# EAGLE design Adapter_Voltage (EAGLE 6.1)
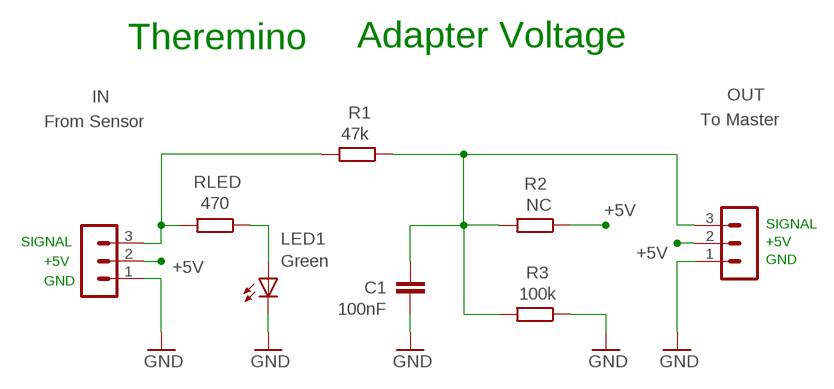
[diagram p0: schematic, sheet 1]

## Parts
C1  100nF  C-EU025-024X044  [C025-024X044]
IN  From Sensor  MA03-1N  [MA03-1]
LED1  Green  LED3MM_F  [LED3MM]
OUT  To Master  MA03-1N  [MA03-1]
R1  47k  R-EU_0204/5  [0204/5]
R2  NC  R-EU_0204/5  [0204/5]
R3  100k  R-EU_0204/5  [0204/5]
RLED  470  R-EU_0204/5  [0204/5]

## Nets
+5V: IN.2 OUT.2 R2.1
GND: C1.2 IN.1 LED1.K(C) OUT.1 R3.1
N$4: LED1.A RLED.1
N$5: C1.1 OUT.3 R1.1 R2.2 R3.2
SIGNAL: IN.3 R1.2 RLED.2

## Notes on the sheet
- Theremino | Adapter Voltage
- SIGNAL
- SIGNAL | +5V
- +5V | GND
- GND

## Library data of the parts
C1 = 00-LIVIO:C-EU: CAPACITOR, European symbol
IN OUT = 03-con-lstb-M:MA03-1: PIN HEADER
LED1 = 00-LIVIO:LED: LEDS
R1-R3 RLED = 00-LIVIO:R-EU_: RESISTOR, European symbol

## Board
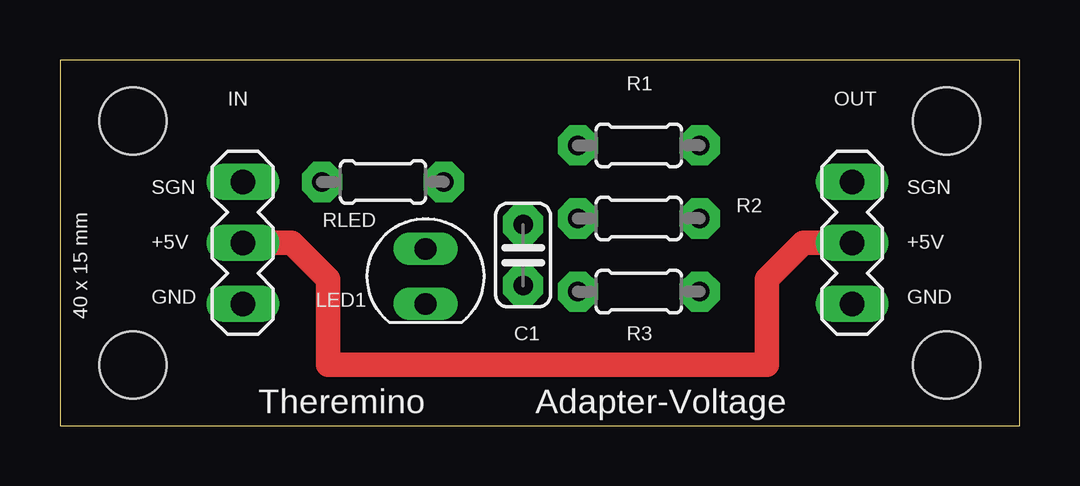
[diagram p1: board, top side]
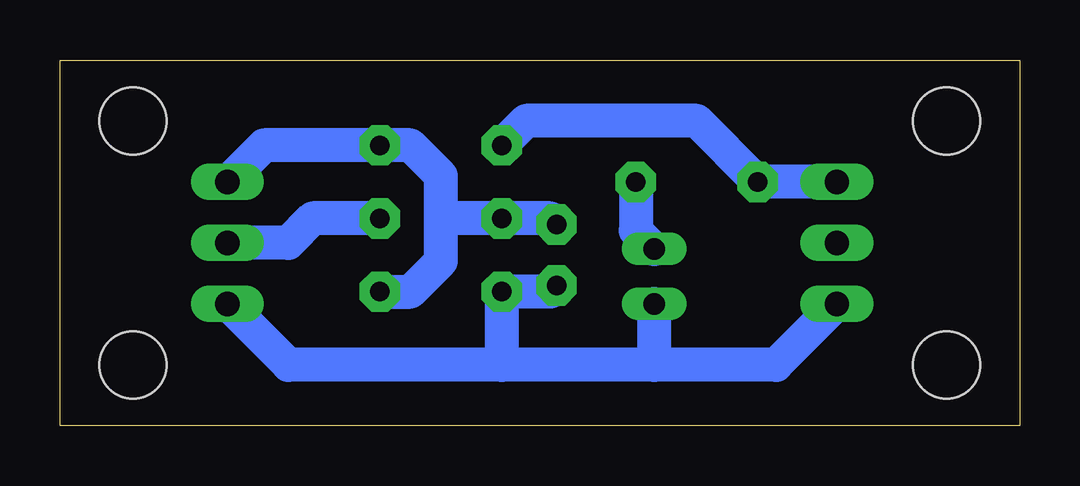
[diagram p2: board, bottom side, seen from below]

Size 40.01 x 15.24 mm. Coordinates in mm from the lower left corner, seen from the top.
Outline: 40.01,15.24 0,15.24 0,0 40.01,0 40.01,15.24
Copper layers (1*16): Top 0.035mm / dielectric 1.5mm / Bottom 0.035mm
Design rules: minimum track width 10mil, minimum drill 31mil, track to track 31mil, track to pad 31mil, pad to pad 31mil, via to via 31mil, smd to smd 31mil, copper to edge 31mil, drill to drill 8mil, minimum pad ring 5mil, minimum via ring 8mil, stop-mask expansion 4mil, vias tented up to drill 0mil, thermal gap 47mil
Holes 2.8 mm at 3.05,2.54 3.05,12.7 36.96,2.54 36.96,12.7

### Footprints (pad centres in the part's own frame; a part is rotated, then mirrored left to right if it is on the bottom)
C025-024X044 = drill 0.813 pad 1.676 octagon: 1 -1.27,0; 2 1.27,0
MA03-1 = drill 1.016 long: 1 -2.54,0; 2 0,0; 3 2.54,0
LED3MM = drill 0.9 long: A -1.016,0; K 1.27,0
0204/5 = drill 0.813 pad 1.676 octagon: 1 -2.54,0; 2 2.54,0

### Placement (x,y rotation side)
C1  19.3,7.11 270 top
IN  7.62,7.62 90 top
LED1  15.24,6.35 270 top
OUT  33.02,7.62 90 top
R1  24.13,11.68 180 top
R2  24.13,8.64 180 top
R3  24.13,5.59 0 top
RLED  13.46,10.16 180 top

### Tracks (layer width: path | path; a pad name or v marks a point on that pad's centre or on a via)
+5V
  Top 1.016: IN.2 9.65,7.62 11.18,6.1 11.18,2.54 29.46,2.54 29.46,6.1 30.99,7.62 OUT.2
  Bottom 1.422: R2.1 29.46,8.64 30.48,7.62 OUT.2
GND
  Bottom 1.422: IN.1 10.16,2.54 15.24,2.54 | 15.24,2.54 21.59,2.54 | 21.59,2.54 30.48,2.54 OUT.1 | LED1.K 15.24,2.54 | C1.2 19.56,5.59 R3.1 21.59,2.54
N$4
  Bottom 1.422: RLED.1 16,8.13 LED1.A
N$5
  Bottom 1.422: OUT.3 31.5,11.68 R1.1 25.4,11.68 24.13,10.41 24.13,8.64 | R3.2 25.4,5.59 24.13,6.86 24.13,8.64 | 24.13,8.64 R2.2 19.56,8.64 C1.1
SIGNAL
  Bottom 1.422: IN.3 RLED.2 13.46,12.7 20.57,12.7 R1.2

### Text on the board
tNames: SGN | SGN | +5V | +5V | GND | GND | 40 x 15 mm | Theremino | Adapter-Voltage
